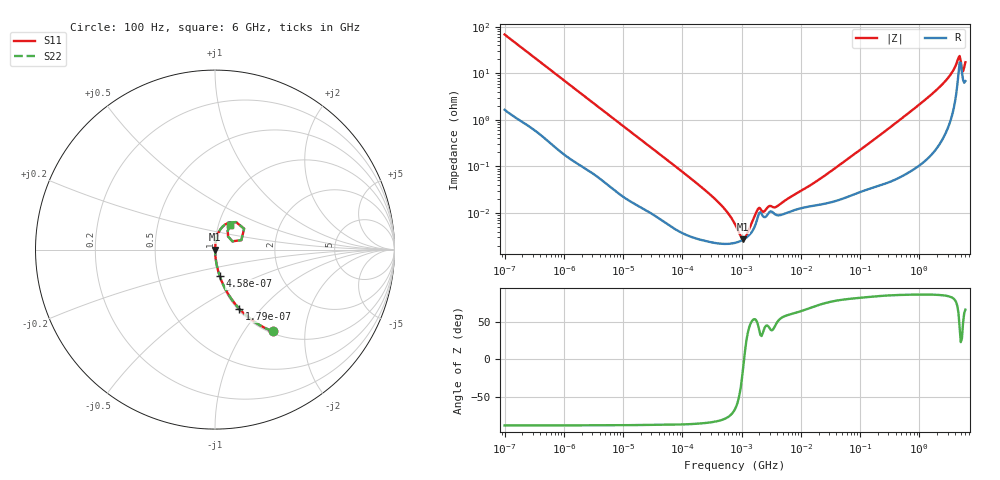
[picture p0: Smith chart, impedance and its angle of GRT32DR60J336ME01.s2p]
!Murata Part Number: GRT32DR60J336ME01
!These Parameters are Measured in Series Mode Connection
!Data Generated on Jun 19, 2026
!  o--ll--o
!Port1  Port2
!  o------o
!Operation Temp=25[degC], DC Bias Voltage=0[V]
!Freq. Start=100[Hz] Stop=6[GHz] 401[Steps]
# Hz S RI R 50
!Freq.(Hz) S11(Real) S11(Imag) S21(Real) S21(Imag) S12(Real) S12(Imag) S22(Real) S22(Imag)
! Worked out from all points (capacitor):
!   401 points, 100 Hz to 6 GHz, reference 50 ohm
!   read as one part in series: C = 23.2 uF near 109 Hz
!   lowest |Z| = 2.72 mohm at 1.06 MHz (marker M1)
!   series resonance near 1.101 MHz, so ESL is about 900 pH
!   S11 on the Smith chart (normalised r, x): 100 Hz: 1.03, -1.37; 179 Hz: 1.02, -0.77; 458 Hz: 1.01, -0.31; 6 GHz: 1.14, +0.32
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100  0.3224 -0.4555  0.6776 0.4555  0.6776 0.4555  0.3224 -0.4555
179  0.1352 -0.3294  0.8648 0.3294  0.8648 0.3294  0.1352 -0.3294
458  0.0267 -0.1482  0.9733 0.1482  0.9733 0.1482  0.0267 -0.1482
2008  0.00227 -0.0356  0.9977 0.0356  0.9977 0.0356  0.00227 -0.0356
40335  8.01e-05 -0.00188  0.9999 0.00188  0.9999 0.00188  8.01e-05 -0.00188
252896  2.49e-05 -0.000294  1 0.000294  1 0.000294  2.49e-05 -0.000294
566185  2.17e-05 -0.000104  1 0.000104  1 0.000104  2.17e-05 -0.000104
774597  2.28e-05 -5.29e-05  1 5.29e-05  1 5.29e-05  2.28e-05 -5.29e-05
1059725  2.66e-05 -5.8e-06  1 5.8e-06  1 5.8e-06  2.66e-05 -5.8e-06
1585629  4.48e-05 6.11e-05  1 -6.11e-05  1 -6.11e-05  4.48e-05 6.11e-05
1983483  9.99e-05 8.2e-05  0.9999 -8.2e-05  0.9999 -8.2e-05  9.99e-05 8.2e-05
2372521  8.2e-05 6.82e-05  0.9999 -6.82e-05  0.9999 -6.82e-05  8.2e-05 6.82e-05
2967816  0.000105 9.49e-05  0.9999 -9.49e-05  0.9999 -9.49e-05  0.000105 9.49e-05
3882480  9.05e-05 0.000102  0.9999 -0.000102  0.9999 -0.000102  9.05e-05 0.000102
1.555665e7  0.000142 0.000394  0.9999 -0.000394  0.9999 -0.000394  0.000142 0.000394
3.124326e8  0.000506 0.0067  0.9995 -0.0067  0.9995 -0.0067  0.000506 0.0067
2.142435e9  0.00523 0.0487  0.9948 -0.0487  0.9948 -0.0487  0.00523 0.0487
3.352442e9  0.0177 0.0901  0.9823 -0.0901  0.9823 -0.0901  0.0177 0.0901
4.385646e9  0.0784 0.1512  0.9216 -0.1512  0.9216 -0.1512  0.0784 0.1512
4.586474e9  0.1178 0.1532  0.8822 -0.1532  0.8822 -0.1532  0.1178 0.1532
5.486059e9  0.0728 0.0732  0.9272 -0.0732  0.9272 -0.0732  0.0728 0.0732
6e9  0.0842 0.1367  0.9158 -0.1367  0.9158 -0.1367  0.0842 0.1367
